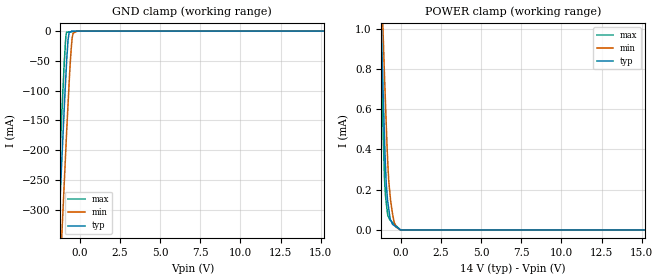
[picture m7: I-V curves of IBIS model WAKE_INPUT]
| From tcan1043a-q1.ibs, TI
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|   WAKE_INPUT Model
[Model]   WAKE_INPUT
Model_type   Input
Vinl = 11
Vinh = 13
|   typ   min   max
C_comp   0.891pF   0.478pF   1.342pF
|  Where Nom  PVT is Nominal Process,   3.3V,  27C
|   Fast PVT is Strong Process,   5.5V, -55C
|   Slow PVT is Weak Process,   2.8V, 150C
[Model spec]
|subparameter
Vinl   11   1.5   37
Vinh   12   2.5   38
[Voltage Range]   14   4.5   40
|Junction Temperature
[Temperature Range]   27   150   -55
[Power Clamp Reference]   14   4.5   40
[GND Clamp Reference]   0   0   0
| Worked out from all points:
|   GND clamp passes 1 mA (typ) near -0.57 V on its own axis
|   POWER clamp passes 1 mA (typ) near -1.20 V on its own axis
[GND Clamp]
|   Voltage   I(typ)   I(min)   I(max)
-14V      -8.504A    -8.611A    -8.439A
-1.487V   -443.6mA   -569.7mA   -364.8mA
-1.345V   -356mA     -483.6mA   -276.6mA
-1.099V   -207.6mA   -334.3mA   -129mA
-880.4mV  -84.6mA    -207.1mA   -15.23mA
-817.4mV  -51.97mA   -170.6mA   -1.706mA
-727.4mV  -14.88mA   -122.9mA   -1.519mA
-660.6mV  -2.452mA   -87.67mA   -1.38mA
-500.4mV  -13.35uA   -19.55mA   -1.047mA
-414.3mV  -8.221uA   -3.718mA   -867.6uA
-174.1mV  -4.22uA    -9.031uA   -367.8uA
28V       0A         0A         -5.859uA
[POWER Clamp]
|   Voltage   I(typ)   I(min)   I(max)
-14V      42.18mA    35.89mA    48mA
-1.325V   1.381mA    1.566mA    1.283mA
-1.204V   1.023mA    1.265mA    859.2uA
-1.099V   713.6uA    1.004mA    520.9uA
-999.7mV  450.5uA    759.6uA    250.3uA
-935mV    308.3uA    616.5uA    163.8uA
-896.6mV  232.2uA    531.5uA    137.5uA
-739mV    104.5uA    244.9uA    62.35uA
-652.6mV  54.48uA    171.3uA    49.21uA
-407.6mV  22.67uA    39.99uA    30.54uA
-6.818mV  359.1nA    141.1nA    0A
28V       0A         0A         0A
